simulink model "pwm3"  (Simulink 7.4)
settings: Solver=ode45  StartTime=0.0  StopTime=.02  MaxStep=1e-6  RelTol=1e-5  AbsTol=1e-5
InitFcn:
  | warning off;fsw=2000
  | Vdc=1
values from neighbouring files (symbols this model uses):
  j = sqrt(-1)    [im3d.m]    (also in imbar1.m; imbarB.m; imchplot66.m; imdef0vec.m)
undefined symbols (not defined in the file or in its folder): fsw
libraries: simulink x5

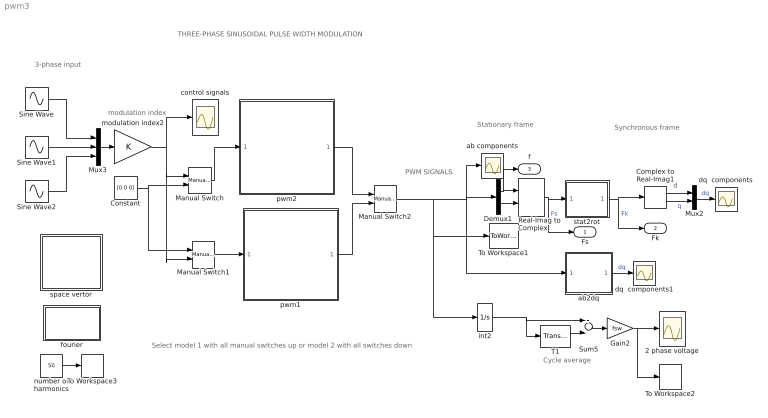
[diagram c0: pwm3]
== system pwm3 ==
  note: THREE-PHASE SINUSOIDAL PULSE WIDTH MODULATION
  note: PWM SIGNALS
  note: Cycle average
  note: modulation index
  note: 3-phase input
  note: d
  note: Stationary frame
  note: Synchronous frame
  note: Select model 1 with all manual switches up or model 2 with all switches down
  2 phase voltage : Scope
  Complex to Real-Imag1 : ComplexToRealImag
  Constant : Constant  Value=[0 0 0]  OutDataType=sfix(16)  OutScaling=2^0
  Demux1 : Demux  Outputs=2
  Gain2 : Gain  Gain=fsw  ParameterDataType=sfix(16)  ParameterScaling=2^0  OutDataType=sfix(16)  OutScaling=2^0
  Manual Switch : simulink/Signal Routing/Manual Switch  SystemSampleTime=-1  sw=1  action=0  varsize=off
  Manual Switch1 : simulink/Signal Routing/Manual Switch  SystemSampleTime=-1  sw=1  action=0  varsize=off
  Manual Switch2 : simulink/Signal Routing/Manual Switch  SystemSampleTime=-1  sw=1  action=0  varsize=off
  Mux2 : Mux  Inputs=2
  Mux3 : Mux  Inputs=3
  Real-Imag to Complex : RealImagToComplex
  Sine Wave : Sin  Amplitude=1  Bias=0  Frequency=2*pi*50  Phase=pi/2  Samples=10  SampleTime=0
  Sine Wave1 : Sin  Amplitude=1  Bias=0  Frequency=2*pi*50  Phase=pi/2 -2*pi/3  Samples=10  SampleTime=0
  Sine Wave2 : Sin  Amplitude=1  Bias=0  Frequency=2*pi*50  Phase=pi/2+2*pi/3  Samples=10  SampleTime=0
  Sum5 : Sum  Inputs=+-  OutDataType=sfix(16)  OutScaling=2^0
  T1 : TransportDelay  DelayTime=1/fsw
  To Workspace1 : ToWorkspace  VariableName=abpwm  SampleTime=-1  SaveFormat=Array
  To Workspace2 : ToWorkspace  VariableName=ab  SampleTime=-1  SaveFormat=Array
  To Workspace3 : ToWorkspace  VariableName=h  SampleTime=-1  SaveFormat=Array
  ab components : Scope
  ab2dq : Subsystem
  control signals : Scope
  dq  components : Scope
  dq  components1 : Scope
  fourier : Subsystem
  int2 : Integrator
  modulation index2 : Gain  ParameterDataType=sfix(16)  ParameterScaling=2^0  OutDataType=sfix(16)  OutScaling=2^0
  number of harmonics : Constant  Value=50  OutDataType=sfix(16)  OutScaling=2^0
  pwm1 : Subsystem
  pwm2 : Subsystem
  space vertor : Subsystem
  stat2rot : Subsystem
  Fs : Outport
  Fk : Outport  Port=2
  f : Outport  Port=3
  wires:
  T1/1 -> Sum5/2
  int2/1 -> Sum5/1, T1/1
  Sum5/1 -> Gain2/1
  Gain2/1 -> 2 phase voltage/1, To Workspace2/1
  pwm2/1(ab) -> Manual Switch2/1
  Sine Wave/1 -> Mux3/1
  Sine Wave1/1 -> Mux3/2
  Sine Wave2/1 -> Mux3/3
  Mux3/1 -> modulation index2/1
  stat2rot/1(rot) -> Complex to Real-Imag1/1, Fk/1  "Fk"
  Real-Imag to Complex/1 -> stat2rot/1(stat), Fs/1  "Fs"
  Mux2/1 -> dq  components/1  "dq"
  Complex to Real-Imag1/1 -> Mux2/1
  Complex to Real-Imag1/2 -> Mux2/2  "q"
  ab2dq/1(dq) -> dq  components1/1  "dq"
  number of harmonics/1 -> To Workspace3/1
  Demux1/1 -> Real-Imag to Complex/1, f/1
  Demux1/2 -> Real-Imag to Complex/2
  modulation index2/1 -> control signals/1, Manual Switch/1, Manual Switch1/2
  pwm1/1(ab) -> Manual Switch2/2
  Manual Switch/1 -> pwm2/1(ABC)
  Constant/1 -> Manual Switch/2, Manual Switch1/1
  Manual Switch1/1 -> pwm1/1(ABC)
  Manual Switch2/1 -> ab components/1, Demux1/1, ab2dq/1(ab), int2/1, To Workspace1/1

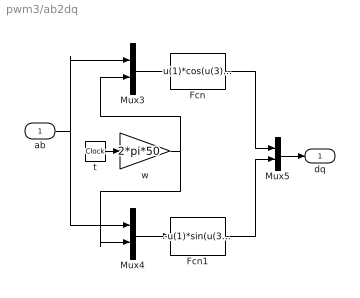
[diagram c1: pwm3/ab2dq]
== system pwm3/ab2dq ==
  ab : Inport  OutDataType=sfix(16)  OutScaling=2^0
  Fcn : Fcn  Expr=u(1)*cos(u(3))+u(2)*sin(u(3))
  Fcn1 : Fcn  Expr=-u(1)*sin(u(3))+u(2)*cos(u(3))
  Mux3 : Mux  Inputs=2
  Mux4 : Mux  Inputs=2
  Mux5 : Mux  Inputs=2
  t : Clock
  w : Gain  Gain=2*pi*50  ParameterDataType=sfix(16)  ParameterScaling=2^0  OutDataType=sfix(16)  OutScaling=2^0
  dq : Outport
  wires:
  t/1 -> w/1
  Mux3/1 -> Fcn/1
  Mux4/1 -> Fcn1/1
  w/1 -> Mux3/2, Mux4/2
  ab/1 -> Mux3/1, Mux4/1
  Fcn1/1 -> Mux5/2
  Fcn/1 -> Mux5/1
  Mux5/1 -> dq/1

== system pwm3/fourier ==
  note: To obtain the Fourier decomposition of a periodic signal: a) run a simulation for one period duration b) Specify the fundamental frequency c) Specify the number of harmonics

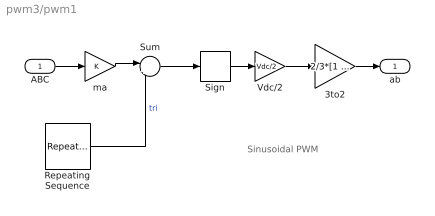
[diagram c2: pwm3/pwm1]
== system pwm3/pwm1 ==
  note: Sinusoidal PWM
  ABC : Inport  OutDataType=sfix(16)  OutScaling=2^0
  3to2 : Gain  Gain=2/3*[1 -0.5 -0.5;0 sqrt(3)/2 -sqrt(3)/2]  Multiplication=Matrix(K*u)  ParameterDataType=sfix(16)  ParameterScaling=2^0  OutDataType=sfix(16)  OutScaling=2^0
  Repeating Sequence : simulink/Sources/Repeating Sequence  SystemSampleTime=-1  rep_seq_t="[0  0.5/fsw 1/fsw]"  rep_seq_y=[1 -1 1]
  Sign : Signum
  Sum : Sum  Inputs=|+-  OutDataType=sfix(16)  OutScaling=2^0
  Vdc/2 : Gain  Gain=Vdc/2  ParameterDataType=sfix(16)  ParameterScaling=2^0  OutDataType=sfix(16)  OutScaling=2^0
  ma : Gain  ParameterDataType=sfix(16)  ParameterScaling=2^0  OutDataType=sfix(16)  OutScaling=2^0
  ab : Outport
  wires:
  ma/1 -> Sum/1
  Sum/1 -> Sign/1
  Repeating Sequence/1 -> Sum/2  "tri"
  Vdc/2/1 -> 3to2/1
  3to2/1 -> ab/1
  ABC/1 -> ma/1
  Sign/1 -> Vdc/2/1

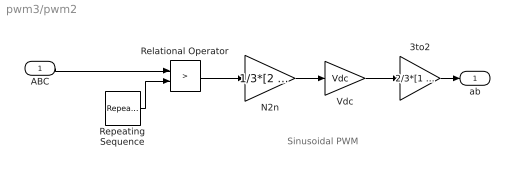
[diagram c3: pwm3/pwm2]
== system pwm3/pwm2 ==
  note: Sinusoidal PWM
  ABC : Inport  OutDataType=sfix(16)  OutScaling=2^0
  3to2 : Gain  Gain=2/3*[1 -0.5 -0.5;0 sqrt(3)/2 -sqrt(3)/2]  Multiplication=Matrix(K*u)  ParameterDataType=sfix(16)  ParameterScaling=2^0  OutDataType=sfix(16)  OutScaling=2^0
  N2n : Gain  Gain=1/3*[2 -1 -1;-1 2 -1;-1 -1 2]  Multiplication=Matrix(K*u)  ParameterDataType=sfix(16)  ParameterScaling=2^0  OutDataType=sfix(16)  OutScaling=2^0
  Relational Operator : RelationalOperator  Operator=>
  Repeating Sequence : simulink/Sources/Repeating Sequence  SystemSampleTime=-1  rep_seq_t="[0  0.5/fsw 1/fsw]"  rep_seq_y=[1 -1 1]
  Vdc : Gain  Gain=Vdc  ParameterDataType=sfix(16)  ParameterScaling=2^0  OutDataType=sfix(16)  OutScaling=2^0
  ab : Outport
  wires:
  ABC/1 -> Relational Operator/1
  3to2/1 -> ab/1
  Relational Operator/1 -> N2n/1
  Repeating Sequence/1 -> Relational Operator/2
  Vdc/1 -> 3to2/1
  N2n/1 -> Vdc/1

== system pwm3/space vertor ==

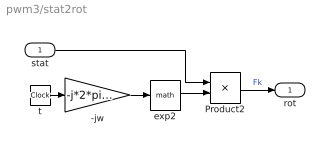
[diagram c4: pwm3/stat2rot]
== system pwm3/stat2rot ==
  stat : Inport  OutDataType=sfix(16)  OutScaling=2^0
  -jw : Gain  Gain=-j*2*pi*50  ParameterDataType=sfix(16)  ParameterScaling=2^0  OutDataType=sfix(16)  OutScaling=2^0
  Product2 : Product  OutDataType=sfix(16)  OutScaling=2^0
  exp2 : Math
  t : Clock
  rot : Outport
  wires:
  exp2/1 -> Product2/2
  -jw/1 -> exp2/1
  t/1 -> -jw/1
  Product2/1 -> rot/1  "Fk"
  stat/1 -> Product2/1
